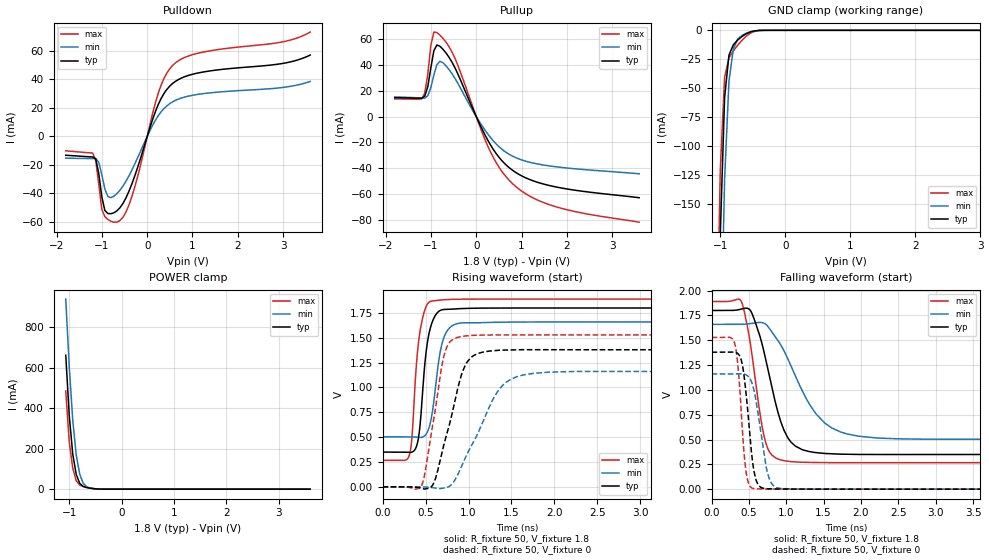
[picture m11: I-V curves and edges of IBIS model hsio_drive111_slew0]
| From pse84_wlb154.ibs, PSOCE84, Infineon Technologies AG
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[Model] hsio_drive111_slew0
Model_type I/O
Enable   Active-High
Vinl  =  0.54
Vinh  =  1.26
Vmeas =  0.9
Cref  =  15pF
| Capacitance   typ   min   max
C_comp   1.183861e-12   1.145095e-12   1.230403e-12
| Variables   typ   min   max
[GND Clamp Reference]   0   0   0
[POWER Clamp Reference]   1.8   1.66   1.89
[Pulldown Reference]   0   0   0
[Pullup Reference]   1.8   1.66   1.89
[Temperature Range]   25   125   -40
[Voltage Range]   1.8   1.66   1.89
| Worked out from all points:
|   slope of the pulldown table from 0 to 0.27 V, typ, clamps not added: 11.2 ohm
|   slope of the pullup table from 0 to 0.27 V, typ, clamps not added: 14.1 ohm
|   GND clamp passes 1 mA (typ) near -0.51 V on its own axis
|   POWER clamp passes 1 mA (typ) near -0.47 V on its own axis
|   falling waveform, R_fixture 50, V_fixture 1.8: 20-80 % time 287ps typ, 483ps min, 189ps max; typ from 1.8 V to 0.349 V
|   falling waveform, R_fixture 50, V_fixture 0: 20-80 % time 108ps typ, 143ps min, 86.4ps max; typ from 1.38 V to 0 V
|   rising waveform, R_fixture 50, V_fixture 1.8: 20-80 % time 94.5ps typ, 112ps min, 86ps max; typ from 0.349 V to 1.8 V
|   rising waveform, R_fixture 50, V_fixture 0: 20-80 % time 237ps typ, 384ps min, 166ps max; typ from 0 V to 1.38 V
[GND Clamp]
| Voltage   I(typ)   I(min)   I(max)
-1.137V   -688mA     -831.1mA   -596.4mA
-1.07V    -398.5mA   -545.5mA   -312.5mA
-1.003V   -176.8mA   -300mA     -120.9mA
-936.6mV  -57.93mA   -128.6mA   -40.51mA
-869.7mV  -21.44mA   -44.12mA   -23.78mA
-802.8mV  -12.54mA   -16.03mA   -17.79mA
-735.9mV  -8.37mA    -7.69mA    -12.93mA
-669mV    -5.28mA    -4.356mA   -8.606mA
-535.2mV  -1.316mA   -1.208mA   -2.332mA
-401.4mV  -73.56uA   -132.2uA   -119.3uA
3.6V      0A         0A         0A
[POWER Clamp]
| Voltage   I(typ)   I(min)   I(max)
-1.07V    662.2mA    940mA      485.7mA
-1.003V   363.7mA    605.6mA    233mA
-936.6mV  172.7mA    341mA      103.9mA
-869.7mV  72.74mA    168.6mA    41.65mA
-802.8mV  28.31mA    73.56mA    19.99mA
-735.9mV  13.11mA    28.55mA    13.36mA
-669mV    7.76mA     11.5mA     8.963mA
-535.2mV  2.357mA    2.863mA    2.668mA
-334.5mV  34.33uA    127.4uA    15.59uA
3.6V      0A         0A         0A
[Pulldown]
| Voltage   I(typ)   I(min)   I(max)
-1.8V     -13.25mA   -15.29mA   -10.11mA
-1.204V   -14.48mA   -15.56mA   -11.72mA
-1.137V   -15.81mA   -15.56mA   -17.11mA
-1.003V   -42.36mA   -26.9mA    -51.24mA
-936.6mV  -52.04mA   -36.88mA   -56.38mA
-869.7mV  -54.22mA   -42.29mA   -58.38mA
-669mV    -52.31mA   -40.21mA   -60.2mA
-401.4mV  -38.39mA   -27.58mA   -48.03mA
248.3mV   22.71mA    14.73mA    30.76mA
558.6mV   37.11mA    24.24mA    49.74mA
1.117V    44.51mA    29.5mA     58.4mA
3.6V      57.13mA    38.61mA    73.29mA
[Pullup]
| Voltage   I(typ)   I(min)   I(max)
-1.8V     14.54mA    15.19mA    13.64mA
-1.204V   14.13mA    14.36mA    13.74mA
-1.137V   15.76mA    14.25mA    18.07mA
-1.07V    23.08mA    16.06mA    32.75mA
-1.003V   37.57mA    22.35mA    54.9mA
-936.6mV  50.85mA    32.04mA    65.25mA
-869.7mV  55.28mA    40.1mA     64.89mA
-468.3mV  37.53mA    29.41mA    44.86mA
310.3mV   -21.62mA   -15.99mA   -26.97mA
806.9mV   -41.6mA    -30.63mA   -51.97mA
1.738V    -54.19mA   -38.68mA   -69.42mA
3.6V      -62.69mA   -44.21mA   -81.58mA
[Ramp]
dV/dt_r   0.827825/0.237045n  0.696274/0.384115n  0.917219/0.166088n
dV/dt_f   0.870357/0.287019n  0.693939/0.482804n  0.973865/0.188685n
R_load = 50
[Falling Waveform]
R_fixture = 50
V_fixture = 1.8
V_fixture_min = 1.66
V_fixture_max = 1.89
| Time   V(typ)   V(min)   V(max)
0s        1.8V       1.66V      1.89V
386.5ps   1.812V     1.66V      1.904V
523.8ps   1.796V     1.668V     1.444V
671.6ps   1.475V     1.678V     651.2mV
750.8ps   1.218V     1.642V     411.8mV
967.2ps   596.9mV    1.397V     287.5mV
1.173ns   413.6mV    1.055V     272.2mV
1.605ns   356.7mV    618.1mV    267.2mV
2.458ns   349mV      507.6mV    266.9mV
50ns      349.4mV    503.4mV    266.9mV
[Falling Waveform]
R_fixture = 50
V_fixture = 0
V_fixture_min = 0
V_fixture_max = 0
| Time   V(typ)   V(min)   V(max)
0s        1.38V      1.16V      1.529V
299.5ps   1.381V     1.16V      1.49V
343.6ps   1.371V     1.161V     1.31V
391.6ps   1.315V     1.162V     854.5mV
471.7ps   889.8mV    1.148V     130.1mV
541.2ps   321.7mV    1.069V     11.16mV
595.1ps   94.18mV    890.5mV    3.312mV
775.2ps   3.126mV    100.1mV    1.057mV
1.034ns   846uV      3.637mV    342.6uV
50ns      10.16nV    819.4nV    3.63nV
[Rising Waveform]
R_fixture = 50
V_fixture = 1.8
V_fixture_min = 1.66
V_fixture_max = 1.89
| Time   V(typ)   V(min)   V(max)
0s        349.4mV    503.4mV    266.9mV
314.8ps   346.2mV    503.5mV    327.7mV
341ps     349.1mV    503.3mV    486.1mV
388.1ps   393.1mV    500mV      1.166V
420.8ps   507.6mV    497.4mV    1.473V
510.7ps   1.386V     535.2mV    1.823V
574.7ps   1.651V     727.2mV    1.87V
678.7ps   1.778V     1.393V     1.881V
788.1ps   1.787V     1.607V     1.887V
50ns      1.8V       1.66V      1.89V
[Rising Waveform]
R_fixture = 50
V_fixture = 0
V_fixture_min = 0
V_fixture_max = 0
| Time   V(typ)   V(min)   V(max)
0s        10.17nV    735.9nV    3.626nV
439.2ps   -10.67mV   -170.8uV   -7.408mV
486ps     -22.39mV   -1.582mV   106.5mV
578.6ps   11.71mV    -7.551mV   599.2mV
747.9ps   533.7mV    -5.696mV   1.408V
933.4ps   1.166V     235.2mV    1.515V
1.144ns   1.351V     607mV      1.528V
1.498ns   1.378V     1.085V     1.529V
2.257ns   1.38V      1.161V     1.529V
50ns      1.38V      1.16V      1.529V
